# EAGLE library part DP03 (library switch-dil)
DIL/CODE SWITCH
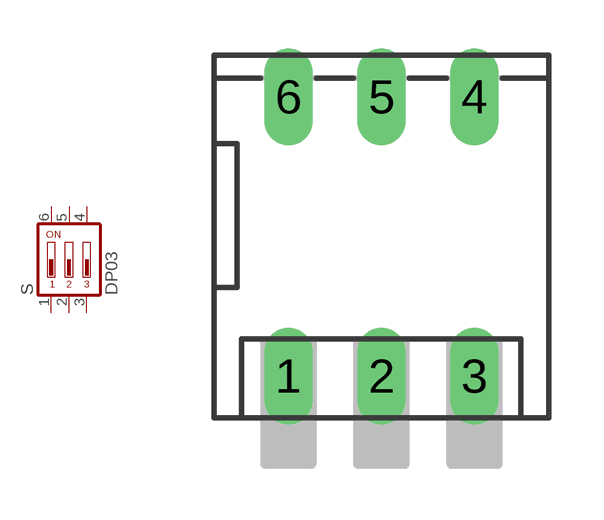
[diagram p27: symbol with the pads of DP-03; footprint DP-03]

Designator prefix S

## DP03 (MPN: MCDP03; OC_FARNELL: 1522004; OC_NEWARK: 74M2976)  [DP-03]
1  1  pas
2  2  pas
3  3  pas
4  4  pas
5  5  pas
6  6  pas

## Footprint DP-03 (pad centres in mm)
DIL/CODE SWITCH
drill 0.813 long: 1 -2.54,-3.81; 2 0,-3.81; 3 2.54,-3.81; 4 2.54,3.81; 5 0,3.81; 6 -2.54,3.81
